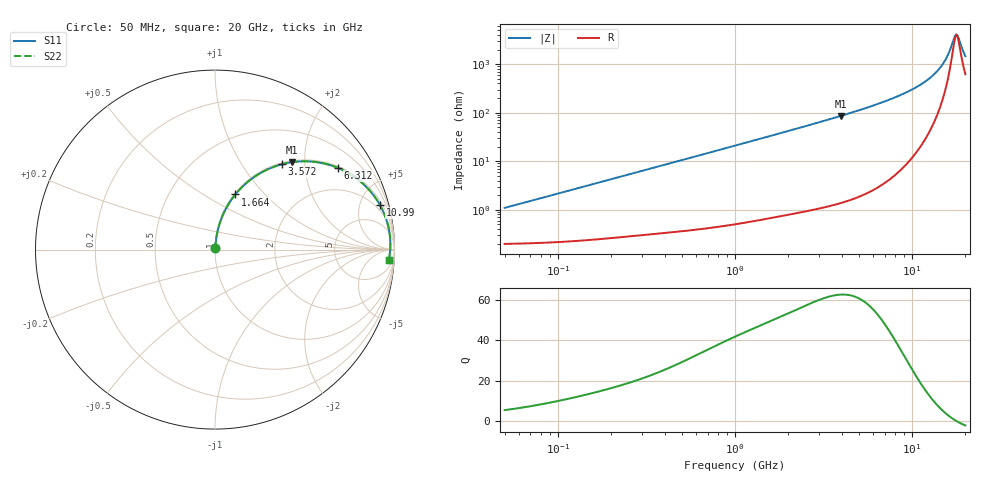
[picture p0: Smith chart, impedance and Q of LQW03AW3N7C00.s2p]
!Murata Part Number: LQW03AW3N7C00
!These Parameters are Measured in Series Mode Connection
!  o--[Z]--o
!Port1  Port2
!  o-------o
!Freq. Start=50[MHz] Stop=20[GHz], 401[Steps]
# Hz S RI R 50
!Freq.(Hz) S11(Real) S11(Imag) S21(Real) S21(Imag) S12(Real) S12(Imag) S22(Real) S22(Imag)
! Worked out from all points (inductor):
!   401 points, 50 MHz to 20 GHz, reference 50 ohm
!   read as one part in series: L = 3.42 nH near 51.52 MHz
!   highest Q = 62.5 at 3.967 GHz (marker M1), where L = 3.46 nH
!   self-resonance near 17.74 GHz
!   S11 on the Smith chart (normalised r, x): 50 MHz: 1.00, +0.02; 1.664 GHz: 1.01, +0.70; 3.572 GHz: 1.02, +1.54; 6.312 GHz: 1.06, +2.97; 10.99 GHz: 1.37, +7.29; 20 GHz: 13, -26
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5e7  0.00209 0.0107  0.9979 -0.0107  0.9979 -0.0107  0.00209 0.0107
1.364002e8  0.00316 0.029  0.9968 -0.029  0.9968 -0.029  0.00316 0.029
3.721004e8  0.00929 0.0775  0.9907 -0.0775  0.9907 -0.0775  0.00929 0.0775
1e9  0.0464 0.1987  0.9536 -0.1987  0.9536 -0.1987  0.0464 0.1987
1.664083e9  0.1133 0.3071  0.8867 -0.3071  0.8867 -0.3071  0.1133 0.3071
2.728004e9  0.254 0.4268  0.746 -0.4268  0.746 -0.4268  0.254 0.4268
3.572216e9  0.3734 0.4757  0.6266 -0.4757  0.6266 -0.4757  0.3734 0.4757
3.967106e9  0.4272 0.4867  0.5728 -0.4867  0.5728 -0.4867  0.4272 0.4867
5.041459e9  0.5599 0.4882  0.4401 -0.4882  0.4401 -0.4882  0.5599 0.4882
6.311513e9  0.6855 0.455  0.3145 -0.455  0.3145 -0.455  0.6855 0.455
7.442007e9  0.7702 0.4096  0.2298 -0.4096  0.2298 -0.4096  0.7702 0.4096
9.178299e9  0.861 0.3303  0.139 -0.3303  0.139 -0.3303  0.861 0.3303
1.098561e10  0.9193 0.2483  0.0807 -0.2483  0.0807 -0.2483  0.9193 0.2483
1.295331e10  0.9552 0.1661  0.0448 -0.1661  0.0448 -0.1661  0.9552 0.1661
1.460232e10  0.9706 0.1041  0.0294 -0.1041  0.0294 -0.1041  0.9706 0.1041
1.573793e10  0.9756 0.065  0.0244 -0.065  0.0244 -0.065  0.9756 0.065
1.621653e10  0.9766 0.0494  0.0234 -0.0494  0.0234 -0.0494  0.9766 0.0494
1.721783e10  0.9769 0.0182  0.0231 -0.0182  0.0231 -0.0182  0.9769 0.0182
1.774144e10  0.9763 0.0027  0.0237 -0.0027  0.0237 -0.0027  0.9763 0.0027
1.828096e10  0.9751 -0.0127  0.0249 0.0127  0.0249 0.0127  0.9751 -0.0127
1.940974e10  0.971 -0.0433  0.029 0.0433  0.029 0.0433  0.971 -0.0433
2e10  0.9681 -0.0585  0.0319 0.0585  0.0319 0.0585  0.9681 -0.0585
